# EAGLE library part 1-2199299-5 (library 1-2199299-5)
TE CONNECTIVITY - 1-2199299-5 - IC SOCKET, DIP, 40POS, TH Source: Datasheet
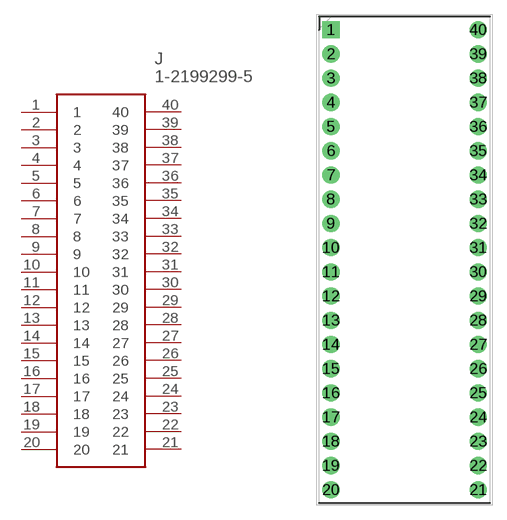
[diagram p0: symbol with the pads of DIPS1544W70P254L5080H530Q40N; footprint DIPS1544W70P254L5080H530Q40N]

Designator prefix J

## 1-2199299-5 (Description: TE CONNECTIVITY - 1-2199299-5 - IC SOCKET, DIP, 40POS, TH; Height: 5.3mm; Manufacturer_Name: TE Connectivity; Manufacturer_Part_Number: 1-2199299-5; Mouser_Part_Number: 571-1-2199299-5; Mouser_Price-Stock: https://www.mouser.co.uk/ProductDetail/TE-Connectivity/1-2199299-5?qs=fK8dlpkaUMthXjoyadQV1Q%3D%3D)  [DIPS1544W70P254L5080H530Q40N]
1  1
2  2
3  3
4  4
5  5
6  6
7  7
8  8
9  9
10  10
11  11
12  12
13  13
14  14
15  15
16  16
17  17
18  18
19  19
20  20
21  21
22  22
23  23
24  24
25  25
26  26
27  27
28  28
29  29
30  30
31  31
32  32
33  33
34  34
35  35
36  36
37  37
38  38
39  39
40  40

## Footprint DIPS1544W70P254L5080H530Q40N (pad centres in mm)
1-2199299-5_A
drill 1.2 pad 1.8 square: 1 0,0
drill 1.2 pad 1.8: 2 0,-2.54; 3 0,-5.08; 4 0,-7.62; 5 0,-10.16; 6 0,-12.7; 7 0,-15.24; 8 0,-17.78; 9 0,-20.32; 10 0,-22.86; 11 0,-25.4; 12 0,-27.94; 13 0,-30.48; 14 0,-33.02; 15 0,-35.56; 16 0,-38.1; 17 0,-40.64; 18 0,-43.18; 19 0,-45.72; 20 0,-48.26; 21 15.44,-48.26; 22 15.44,-45.72; 23 15.44,-43.18; 24 15.44,-40.64; 25 15.44,-38.1; 26 15.44,-35.56; 27 15.44,-33.02; 28 15.44,-30.48; 29 15.44,-27.94; 30 15.44,-25.4; 31 15.44,-22.86; 32 15.44,-20.32; 33 15.44,-17.78; 34 15.44,-15.24; 35 15.44,-12.7; 36 15.44,-10.16; 37 15.44,-7.62; 38 15.44,-5.08; 39 15.44,-2.54; 40 15.44,0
